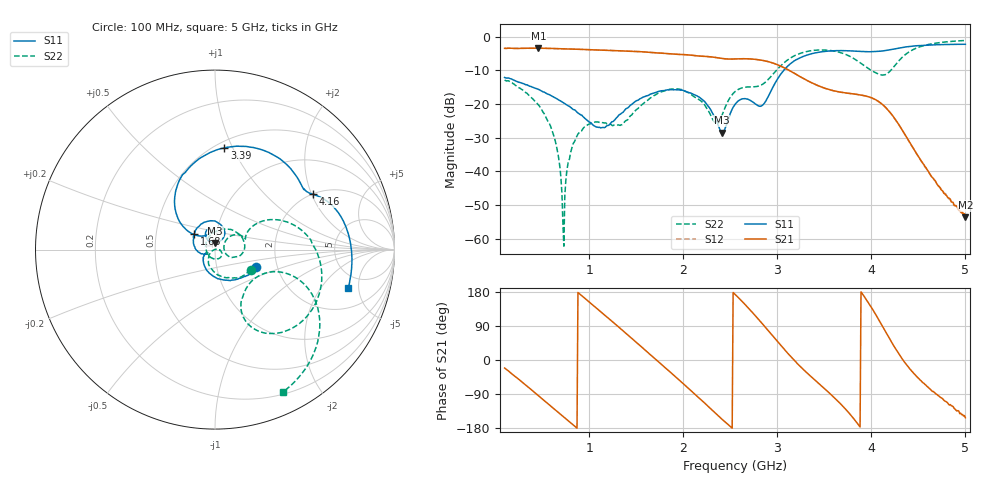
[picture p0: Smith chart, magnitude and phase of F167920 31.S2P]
!  2-Port S-parameters saved by WinCal
! VAR MeasName=S-Parameters (CALIBRATED_DATA) read from VNA (N5242A)
! VAR MeasDate=2016-11-22 9:56:41
! VAR NAME=F167920 31
! VAR FILENAME=F167920 31.S2P
! VAR DATE=2016-11-22 9:56:41
! VAR PHYS_PORTS=1,2
# Hz S DB R 50
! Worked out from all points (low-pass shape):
!   491 points, 100 MHz to 5 GHz, reference 50 ohm
!   highest |S21| = -3.40 dB at 460 MHz (marker M1); lowest = -53.7 dB at 5 GHz (marker M2)
!   |S21| within 3 dB of the highest: start of sweep to 2.398 GHz
!   lowest |S11| = -28.5 dB at 2.41 GHz (marker M3), VSWR 1.08, Z = 50 + j3.77 ohm
!   |S11| at or under -10 dB: start of sweep to 3.068 GHz
!   |S22| runs from -62.3 to -1.1 dB; largest |S21 - S12| = 0.0012
!   S11 on the Smith chart (normalised r, x): 100 MHz: 1.55, -0.32; 1.68 GHz: 0.78, +0.14; 3.39 GHz: 0.55, +0.93; 4.16 GHz: 2.01, +2.04; 5 GHz: 3.64, -3.81
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1e8  -12.11 -22.8  -3.46 -21.2  -3.46 -21.2  -12.86 -29.2
4.6e8  -15.65 -83.1  -3.40 -94.3  -3.40 -94.2  -20.27 -108.3
6.4e8  -18.19 -112.5  -3.53 -132.0  -3.52 -132.0  -31.16 -148.5
6.8e8  -18.87 -118.6  -3.57 -140.3  -3.56 -140.2  -37.09 -158.0
7.2e8  -19.53 -124.8  -3.60 -148.5  -3.60 -148.5  -55.60 -160.4
7.9e8  -20.69 -135.7  -3.64 -163.1  -3.64 -163.1  -36.36 3.7
9.2e8  -23.30 -152.8  -3.76 169.8  -3.76 169.8  -27.95 -25.1
1.3e9  -23.81 -155.1  -4.17 89.8  -4.17 89.8  -26.26 -155.3
1.68e9  -16.81 143.8  -4.73 7.4  -4.72 7.4  -17.68 61.4
1.74e9  -16.26 133.3  -4.85 -5.5  -4.85 -5.6  -16.69 47.7
2.08e9  -16.74 79.0  -5.48 -80.6  -5.48 -80.6  -17.06 -15.1
2.41e9  -28.49 87.4  -6.45 -155.9  -6.45 -155.9  -23.49 35.5
2.55e9  -20.15 122.8  -6.61 173.4  -6.61 173.3  -16.33 33.1
2.86e9  -19.87 131.9  -7.12 90.0  -7.12 89.9  -13.82 28.0
3.08e9  -9.62 132.7  -9.33 26.2  -9.34 26.1  -7.55 22.1
3.37e9  -5.02 87.4  -13.75 -46.4  -13.77 -46.5  -4.11 -18.0
3.39e9  -4.90 84.8  -14.03 -50.8  -14.04 -50.9  -4.05 -20.6
3.71e9  -4.15 50.8  -16.63 -125.5  -16.67 -125.3  -5.08 -57.1
4.16e9  -4.06 29.5  -21.26 70.6  -21.29 70.8  -11.11 -33.6
4.19e9  -3.92 28.4  -22.17 57.6  -22.21 57.8  -10.48 -27.0
4.5e9  -2.65 11.0  -35.59 -48.1  -35.58 -48.0  -3.16 -33.1
5e9  -2.25 -15.9  -53.67 -152.3  -53.74 -151.2  -1.11 -64.5
